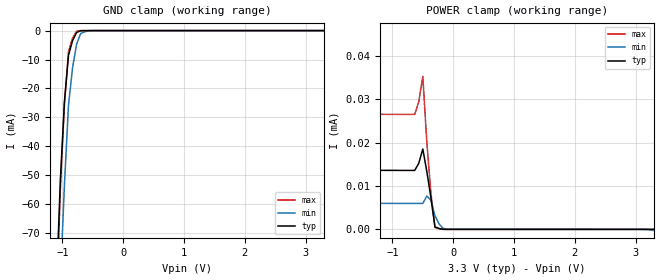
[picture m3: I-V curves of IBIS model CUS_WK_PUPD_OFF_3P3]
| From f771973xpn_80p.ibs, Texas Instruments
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|CUS_WK_PD_ON_3P3; WEAK_PULLDOWN_ON
|   Model Cell CUS_WK_PUPD_OFF_3P3
|CUS_WK_PUPD_OFF_3P3
[Model]   CUS_WK_PUPD_OFF_3P3
Model_type   Input
Polarity   Non-Inverting
Vinl =  0.8
Vinh =  2
C_comp   2.12034p   1.0392p   2.53442p
[Model Spec]
Vinl   0.8   0.8   0.8
Vinh   2   2   2
[Temperature Range]   25   155   -40
[Voltage Range]   3.3   2.97   3.63
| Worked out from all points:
|   GND clamp passes 1 mA (typ) near -0.78 V on its own axis
| Nom Voltages:
|   BIASFET=3.3, VDD=1.2, VDDS=3.3, VSS=0
| Min Voltages:
|   BIASFET=2.97, VDD=1.08, VDDS=2.97, VSS=0
| Max Voltages:
|   BIASFET=3.63, VDD=1.32, VDDS=3.63, VSS=0
[POWER_clamp]
|   voltage   I(typ)   I(min)   I(max)
-3.3V     150.5uA    636.5mA    31.16uA
-3.233V   62.15uA    593.8mA    30.78uA
-3.167V   17uA       551.3mA    30.41uA
-3.1V     15.04uA    508.8mA    30.07uA
-1.967V   13.75uA    47.6uA     26.93uA
-1.9V     13.73uA    10.08uA    26.86uA
-1.767V   13.68uA    6.22uA     26.75uA
-633.3mV  13.58uA    5.976uA    26.46uA
-500mV    18.5uA     5.973uA    35.23uA
-366.7mV  7.288uA    6.734uA    8.322uA
-300mV    565.8nA    3.113uA    435.6nA
3.3V      -83.44pA   -266.7nA   -87.08pA
[GND_clamp]
|   voltage   I(typ)   I(min)   I(max)
-3.3V     -2.204A    -1.834A    -3.186A
-1.1V     -88.83mA   -124.4mA   -95.53mA
-1.033V   -51.35mA   -86.05mA   -54.49mA
-966.7mV  -24.58mA   -53.16mA   -25.05mA
-900mV    -8.508mA   -25.71mA   -7.216mA
-833.3mV  -3.462mA   -12.88mA   -2.621mA
-766.7mV  -641.8uA   -4.656mA   -220uA
-700mV    -47.87uA   -1.025mA   -14.14uA
-566.7mV  -3.25uA    -83.32uA   -2.52uA
3.3V      757.1pA    5.854uA    409.8pA
